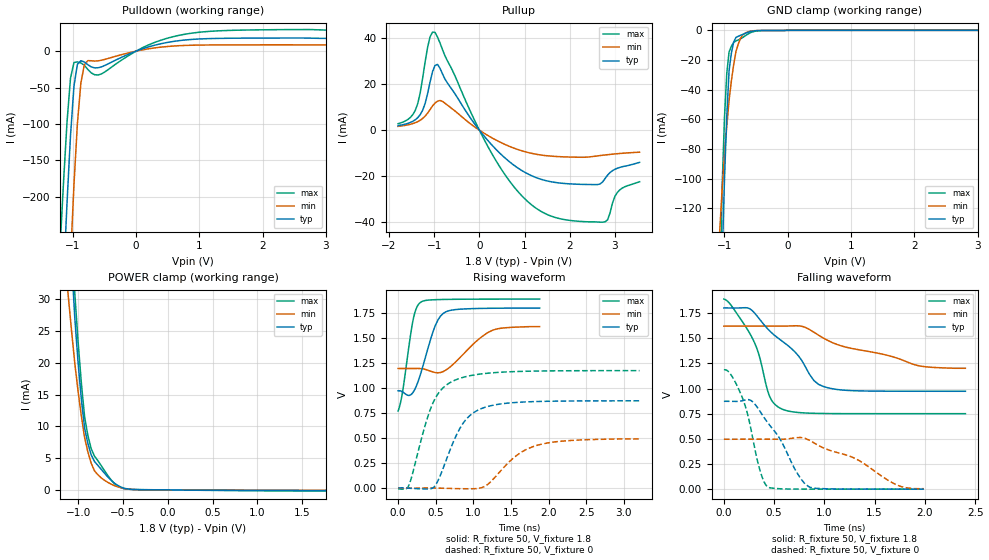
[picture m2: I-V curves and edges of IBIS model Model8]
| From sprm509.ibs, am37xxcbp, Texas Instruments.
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| Model based on original model for BQ1850OMAPSMART2HYFBPB_SSBHH
|   Sub model T2HYFBPB_H50_1_PU1_1P8
[model]   Model8
|[Input Load]   PU
|[Output Drive] LB1
|Voltage   1.8V
|Mode   I/O
Model_type   I/O
Polarity   Non-Inverting
Enable   Active-Low
Vinl =  0.63
Vinh =  1.17
Cref =  15pF
Rref =  100.0000M
Vref =  0V
Vmeas =  0.9
C_comp   1.383404p   1.221591p   1.559603p
[Model Spec]
Vinl   0.63   0.567   0.6615
Vinh   1.17   1.053   1.2285
[Temperature Range]   25   125   -40
[Voltage Range]   1.8   1.62   1.89
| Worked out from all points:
|   slope of the pulldown table from 0 to 0.27 V, typ, clamps not added: 35.5 ohm
|   slope of the pullup table from 0 to 0.27 V, typ, clamps not added: 42.9 ohm
|   GND clamp passes 1 mA (typ) near -0.60 V on its own axis
|   POWER clamp passes 1 mA (typ) near -0.59 V on its own axis
|   rising waveform, R_fixture 50, V_fixture 1.8: 20-80 % time 203ps typ, 355ps min, 130ps max; typ from 0.973 V to 1.8 V
|   rising waveform, R_fixture 50, V_fixture 0: 20-80 % time 331ps typ, 447ps min, 306ps max; typ from 0.001 V to 0.873 V
|   falling waveform, R_fixture 50, V_fixture 1.8: 20-80 % time 455ps typ, 839ps min, 249ps max; typ from 1.8 V to 0.974 V
|   falling waveform, R_fixture 50, V_fixture 0: 20-80 % time 311ps typ, 591ps min, 178ps max; typ from 0.874 V to 0.002 V
[POWER_clamp]
-1.8V     290.9mA    160.5mA    340.9mA
-1.109V   45.83mA    30.44mA    51.29mA
-1.073V   36.05mA    25.03mA    40.56mA
-1.036V   26.99mA    19.89mA    30.86mA
-963.6mV  14.28mA    11.63mA    16.86mA
-927.3mV  9.746mA    8.243mA    11.5mA
-890.9mV  7.306mA    5.98mA     8.567mA
-818.2mV  4.49mA     3.024mA    5.342mA
-672.7mV  2.114mA    1.23mA     2.346mA
-563.6mV  762.3uA    511.4uA    680.1uA
-418.2mV  103.6uA    97.29uA    94.35uA
1.764V    -96.73uA   -46.45uA   -163.5uA
[Pulldown]
-1.8V     -1.423A    -2.058A    -1.157A
-1.2V     -415.4mA   -653.2mA   -267mA
-1.145V   -309.6mA   -525.9mA   -177.9mA
-1.091V   -207.6mA   -402.8mA   -96.72mA
-1.036V   -115.8mA   -286.9mA   -37.04mA
-981.8mV  -48.02mA   -183.2mA   -15.64mA
-927.3mV  -18.04mA   -99.43mA   -14.72mA
-872.7mV  -13.22mA   -44mA      -16.16mA
-763.6mV  -18.5mA    -13.02mA   -24.96mA
-545.5mV  -21.5mA    -12.44mA   -31.16mA
872.7mV   16.04mA    8.112mA    24.59mA
3.545V    17.47mA    8.568mA    28.69mA
[Pullup]
-1.8V     2.003mA    1.674mA    2.831mA
-1.418V   4.544mA    3.255mA    8.658mA
-1.255V   8.732mA    5.125mA    22.8mA
-1.091V   20.98mA    8.984mA    40.62mA
-981.8mV  28.13mA    11.78mA    42.49mA
-818.2mV  24.52mA    12.54mA    35.08mA
272.7mV   -6.354mA   -3.271mA   -10.08mA
1.2V      -20.15mA   -10.23mA   -33.12mA
1.8V      -22.99mA   -11.52mA   -38.52mA
2.782V    -21mA      -10.76mA   -39.77mA
3.055V    -16.52mA   -10.21mA   -26.99mA
3.545V    -13.98mA   -9.552mA   -22.39mA
[GND_clamp]
-1.8V     -2.709A    -1.157A    -3.075A
-1.073V   -228.8mA   -133.6mA   -187.2mA
-1.036V   -154.6mA   -106.9mA   -104.7mA
-1V       -100.5mA   -84.7mA    -59.14mA
-963.6mV  -58.02mA   -64.83mA   -29.09mA
-927.3mV  -27.26mA   -47.26mA   -14.57mA
-890.9mV  -15.37mA   -34.15mA   -10.73mA
-854.5mV  -7.879mA   -23.16mA   -8.224mA
-818.2mV  -4.778mA   -14.29mA   -7.06mA
-709.1mV  -2.726mA   -2.962mA   -4.785mA
-527.3mV  -381uA     -250uA     -722.9uA
3.6V      0A         0A         0A
[Ramp]
dV/dt_f  0.4976841/0.4560859n  0.2563561/0.8513039n  0.6841951/0.2501823n
dV/dt_r  0.5290636/0.3321713n  0.3018805/0.4610803n  0.7108378/0.3061483n
R_load = 50
[Rising Waveform]
R_fixture = 50
V_fixture = 1.8
V_fixture_min = 1.62
V_fixture_max = 1.89
0s        973.4mV    1.196V     770.9mV
56ps      964.1mV    1.196V     946mV
144.8ps   927.1mV    1.196V     1.42V
208ps     967.3mV    1.196V     1.71V
253.6ps   1.04V      1.196V     1.815V
299.2ps   1.142V     1.195V     1.857V
487.2ps   1.61V      1.156V     1.883V
627.2ps   1.759V     1.176V     1.886V
1.238ns   1.798V     1.572V     1.889V
1.882ns   1.8V       1.614V     1.89V
[Rising Waveform]
R_fixture = 50
V_fixture = 0
V_fixture_min = 0
V_fixture_max = 0
0s        1.435mV    1.376mV    -6.315mV
152.8ps   -367.5uV   715.5uV    44.39mV
371.2ps   -8.275mV   2.387mV    656.7mV
473.6ps   8.928mV    1.902mV    867.4mV
717.6ps   431.6mV    -2.859mV   1.066V
912ps     694.6mV    -5.564mV   1.117V
1.238ns   824.9mV    68.63mV    1.152V
1.563ns   856.5mV    319.8mV    1.165V
1.85ns    866.1mV    428.8mV    1.171V
3.21ns    873.1mV    491.9mV    1.175V
[Falling Waveform]
R_fixture = 50
V_fixture = 1.8
V_fixture_min = 1.62
V_fixture_max = 1.89
0s        1.8V       1.62V      1.889V
270.4ps   1.784V     1.62V      1.525V
342.4ps   1.705V     1.62V      1.358V
453.6ps   1.575V     1.62V      925.5mV
579.2ps   1.471V     1.62V      796.5mV
745.6ps   1.32V      1.622V     762.4mV
896.8ps   1.079V     1.559V     754.8mV
1.035ns   1.008V     1.477V     752.5mV
1.931ns   973.7mV    1.229V     751mV
2.404ns   973.5mV    1.202V     751mV
[Falling Waveform]
R_fixture = 50
V_fixture = 0
V_fixture_min = 0
V_fixture_max = 0
0s        874mV      497.5mV    1.187V
72ps      873.5mV    497.3mV    1.135V
186.4ps   880.3mV    498.1mV    902.4mV
272ps     880.2mV    498.2mV    584.1mV
362.4ps   769.7mV    498.1mV    177mV
437.6ps   659.8mV    497.9mV    23.32mV
852ps     22.21mV    487mV      2.579mV
1.298ns   2.354mV    310.3mV    2.371mV
1.721ns   1.987mV    43.91mV    2.357mV
1.989ns   1.929mV    6.867mV    2.356mV
